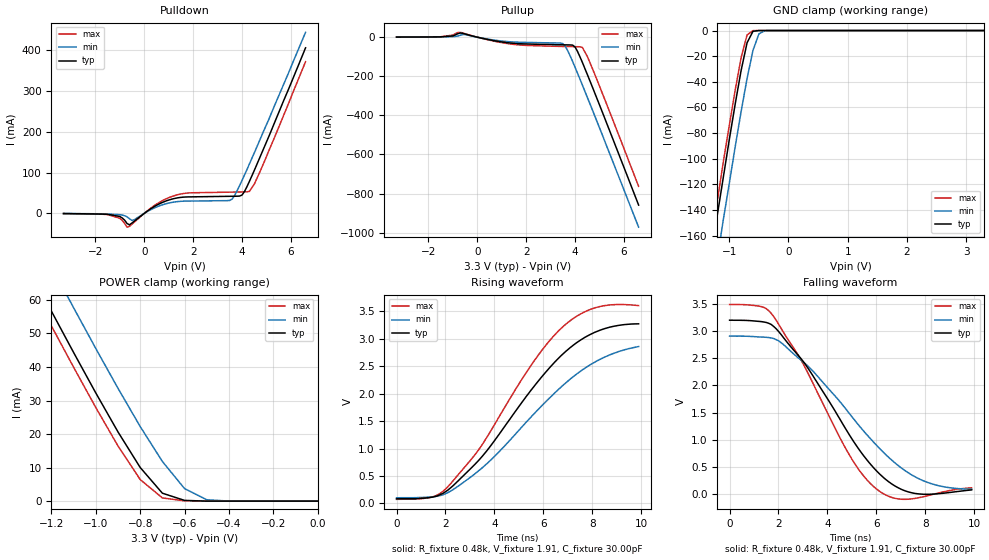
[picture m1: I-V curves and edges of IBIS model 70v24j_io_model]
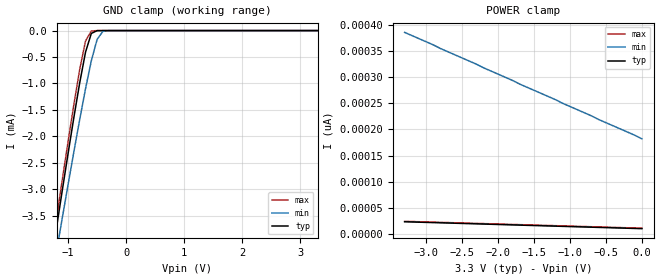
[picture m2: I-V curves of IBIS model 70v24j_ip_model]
| IBIS file 70v24j.ibs created by s2ibis2 version 1.0
| North Carolina State University Electronics Research Laboratory  1995
[IBIS ver]   2.1
[File name]   70v24j.ibs
[File Rev]   3.2
[Date]   11/11/04
[Source]   Integrated Device Technology, Inc.
[Notes]   1.Temperatures: typ=25C, min=100C, max=0C 2.Cemos7_5v process.
   3.RRmp rates based on 50 ohm load.
   IO & IP models corrected.  TH 11/11/04
[Disclaimer]   This information is for modeling purpose only, and is not
   guaranteed.
[Copyright]   Copyright 1997, Integrated Device Technology, Inc. all rights
   reserved
|   Component idt70v24
[Component]   idt70v24
[Manufacturer]   Integrated Device Technology
[Package]
| variable   typ   min   max
R_pkg   100.00m   50.00m   0.15
L_pkg   12.00nH   11.00nH   13.00nH
C_pkg   0.80pF   0.70pF   0.90pF
[Pin]  signal_name   model_name   R_pin   L_pin   C_pin
1   VCC   POWER
2   OEBL   70v24j_ip_model
3   IO0L   70v24j_io_model
4   IO1L   70v24j_io_model
5   GND   GND
6   IO2L   70v24j_io_model
7   IO3L   70v24j_io_model
8   IO4L   70v24j_io_model
9   IO5L   70v24j_io_model
10   IO6L   70v24j_io_model
11   IO7L   70v24j_io_model
12   IO8L   70v24j_io_model
13   IO9L   70v24j_io_model
14   IO10L   70v24j_io_model
15   IO11L   70v24j_io_model
16   IO12L   70v24j_io_model
17   IO13L   70v24j_io_model
18   GND   GND
19   IO14L   70v24j_io_model
20   IO15L   70v24j_io_model
21   VCC   POWER
22   GND   GND
23   IO0R   70v24j_io_model
24   IO1R   70v24j_io_model
25   IO2R   70v24j_io_model
26   VCC   POWER
27   IO3R   70v24j_io_model
28   IO4R   70v24j_io_model
29   IO5R   70v24j_io_model
30   IO6R   70v24j_io_model
31   IO7R   70v24j_io_model
32   IO8R   70v24j_io_model
33   IO9R   70v24j_io_model
34   IO10R   70v24j_io_model
35   IO11R   70v24j_io_model
36   IO12R   70v24j_io_model
37   IO13R   70v24j_io_model
38   IO14R   70v24j_io_model
39   GND   GND
40   IO15R   70v24j_io_model
41   OEBR   70v24j_ip_model
42   RWBR   70v24j_ip_model
43   GND   GND
44   SEMBR   70v24j_ip_model
45   CEBR   70v24j_ip_model
46   UBR   70v24j_ip_model
47   LBR   70v24j_ip_model
48   A12R   70v24j_ip_model
49   A11R   70v24j_ip_model
50   A10R   70v24j_ip_model
51   A9R   70v24j_ip_model
52   A8R   70v24j_ip_model
53   A7R   70v24j_ip_model
54   A6R   70v24j_ip_model
55   A5R   70v24j_ip_model
56   A4R   70v24j_ip_model
57   A3R   70v24j_ip_model
58   A2R   70v24j_ip_model
59   A1R   70v24j_ip_model
60   A0R   70v24j_ip_model
61   INTBR   70v24j_ip_model
62   BUSYBR   70v24j_io_model
63   MSBR   70v24j_ip_model
64   GND   GND
65   BUSYBL   70v24j_io_model
66   INTBL   70v24j_ip_model
67   A0L   70v24j_ip_model
68   A1L   70v24j_ip_model
69   A2L   70v24j_ip_model
70   A3L   70v24j_ip_model
71   A4L   70v24j_ip_model
72   A5L   70v24j_ip_model
73   A6L   70v24j_ip_model
74   A7L   70v24j_ip_model
75   A8L   70v24j_ip_model
76   A9L   70v24j_ip_model
77   A10L   70v24j_ip_model
78   A11L   70v24j_ip_model
79   A12L   70v24j_ip_model
80   LBL   70v24j_ip_model
81   UBL   70v24j_ip_model
82   CEBL   70v24j_ip_model
83   SEMBL   70v24j_ip_model
84   RWBL   70v24j_ip_model
| Models and submodels in the file (2): 70v24j_io_model (I/O), 70v24j_ip_model (Input)
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| in   in   dummy_model
| oel  oel   dummy_model
|   Model 70v24j_io_model
[Model]   70v24j_io_model
Model_type   I/O
Polarity   Non-Inverting
Enable   Active-High
Vinl =  0.800V
Vinh =  2.000V
Vmeas =  1.500V
C_comp   3.00pF   NA   NA
[Temperature Range]   25.00   100.00   0.000
[Voltage Range]   3.30V   3.00V   3.60V
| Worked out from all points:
|   slope of the pulldown table from 0 to 0.495 V, typ, clamps not added: 25.2 ohm
|   slope of the pullup table from 0 to 0.495 V, typ, clamps not added: 36.8 ohm
|   GND clamp passes 1 mA (typ) near -0.60 V on its own axis
|   POWER clamp passes 1 mA (typ) near -0.64 V on its own axis
|   rising waveform, R_fixture 0.48k, V_fixture 1.91, C_fixture 30.00pF: 20-80 % time 3.38ns typ, 3.7ns min, 3.12ns max; typ from 0.085 V to 3.27 V
|   falling waveform, R_fixture 0.48k, V_fixture 1.91, C_fixture 30.00pF: 20-80 % time 2.73ns typ, 3.33ns min, 2.38ns max; typ from 3.21 V to 0.072 V
[Pulldown]
| voltage   I(typ)   I(min)   I(max)
-3.3V     -300uA     -100uA     -400uA
-1.5V     -2.1mA     -1.4mA     -2.7mA
-1V       -7.34mA    -3mA       -11.82mA
-700mV    -24.76mA   -8.36mA    -33.61mA
-500mV    -23.52mA   -17.09mA   -26.24mA
400mV     16.4mA     13.1mA     18.68mA
1.2V      36.14mA    27.71mA    42.98mA
3.6V      42.09mA    35.54mA    52.29mA
4V        45.03mA    80.8mA     52.68mA
4.3V      78.13mA    121mA      54.03mA
4.5V      105mA      148mA      71.43mA
6.6V      406mA      444mA      372mA
[Pullup]
| voltage   I(typ)   I(min)   I(max)
-3.3V     500uA      600uA      600uA
-1.5V     1.64mA     1.1mA      1.95mA
-1V       6.29mA     2.68mA     10.62mA
-700mV    21.31mA    9.36mA     24.78mA
-500mV    16.4mA     13.61mA    17.88mA
1.3V      -29.2mA    -23.2mA    -33.88mA
3.5V      -39.14mA   -32.8mA    -47.46mA
3.7V      -39.55mA   -69.14mA   -47.96mA
4V        -50.05mA   -154mA     -48.63mA
4.3V      -129mA     -245mA     -52.79mA
4.5V      -190mA     -307mA     -97.94mA
6.6V      -859mA     -972mA     -763mA
[GND_clamp]
| voltage   I(typ)   I(min)   I(max)
-3.3V     -782mA     -813mA     -772mA
-1.3V     -172mA     -206mA     -161mA
-1.2V     -143mA     -177mA     -132mA
-1.1V     -114mA     -147mA     -102mA
-1V       -84.95mA   -119mA     -73.85mA
-900mV    -57.1mA    -90.38mA   -46.23mA
-800mV    -30.99mA   -63.03mA   -21.01mA
-700mV    -9.534mA   -37.37mA   -3.418mA
-600mV    -615uA     -15.47mA   -80.43uA
-500mV    -13.71uA   -2.616mA   -1.165uA
-400mV    -280nA     -145uA     -16.67nA
3.3V      38.75pA    737nA      37.71pA
[POWER_clamp]
| voltage   I(typ)   I(min)   I(max)
-3.3V     327mA      340mA      323mA
-1.3V     69.13mA    82.47mA    64.73mA
-1.2V     56.64mA    70mA       52.24mA
-1.1V     44.32mA    57.67mA    39.93mA
-1V       32.26mA    45.51mA    27.91mA
-900mV    20.65mA    33.65mA    16.46mA
-800mV    10.05mA    22.26mA    6.453mA
-700mV    2.37mA     11.84mA    958uA
-600mV    220uA      3.738mA    89.37uA
-500mV    1.528uA    408uA      130nA
-400mV    31.23nA    16.43uA    1.901nA
0V        38.73pA    1.793nA    42.34pA
[Ramp]
| variable   typ   min   max
dV/dt_r   0.97/2.56n   0.75/2.76n   1.16/2.41n
dV/dt_f   1.14/2.25n   0.88/2.68n   1.36/1.86n
R_load = 50.00
[Rising Waveform]
R_fixture = 0.48k
V_fixture = 1.91
C_fixture = 30.00pF
R_dut = 100.00m
L_dut = 4.00nH
C_dut = 10.00pF
| time   V(typ)   V(min)   V(max)
0s        84.6mV     104mV      75.61mV
1.4ns     111mV      119mV      112mV
2.1ns     244mV      197mV      306mV
3.4ns     806mV      611mV      1.005V
5.8ns     2.231V     1.716V     2.704V
6.4ns     2.541V     1.983V     3.037V
7ns       2.8V       2.226V     3.294V
7.6ns     2.997V     2.433V     3.469V
8.3ns     3.152V     2.62V      3.585V
9.9ns     3.272V     2.858V     3.604V
[Falling Waveform]
R_fixture = 0.48k
V_fixture = 1.91
C_fixture = 30.00pF
R_dut = 100.00m
L_dut = 4.00nH
C_dut = 10.00pF
| time   V(typ)   V(min)   V(max)
0s        3.205V     2.912V     3.495V
1.2ns     3.183V     2.896V     3.466V
1.7ns     3.127V     2.878V     3.333V
3.1ns     2.389V     2.401V     2.322V
5ns       1.016V     1.425V     641mV
6.1ns     382mV      854mV      57.18mV
6.8ns     135mV      557mV      -86.2mV
7.5ns     13.93mV    336mV      -90.56mV
8.5ns     126uV      155mV      10.6mV
9.9ns     71.96mV    85.36mV    111mV
|   Model 70v24j_ip_model
[Model]   70v24j_ip_model
Model_type   Input
Vinl =  0.800V
Vinh =  2.000V
Vmeas =  1.500V
C_comp   3.00pF   NA   NA
[Temperature Range]   25.00   100.00   0.000
[Voltage Range]   3.30V   3.00V   3.60V
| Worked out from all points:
|   GND clamp passes 1 mA (typ) near -0.80 V on its own axis
[GND_clamp]
| voltage   I(typ)   I(min)   I(max)
-3.3V     -19.14mA   -18.01mA   -19.55mA
-1.3V     -4.44mA    -4.817mA   -4.291mA
-1.2V     -3.724mA   -4.175mA   -3.549mA
-1.1V     -3.016mA   -3.537mA   -2.815mA
-900mV    -1.636mA   -2.286mA   -1.391mA
-800mV    -986uA     -1.68mA    -732uA
-700mV    -408uA     -1.1mA     -197uA
-600mV    -53.66uA   -571uA     -7.707uA
-500mV    -1.345uA   -166uA     -115nA
-400mV    -27.62nA   -13.71uA   -1.646nA
-200mV    -15.59pA   -29nA      -4.735pA
3.3V      9.916pA    201pA      9.6pA
[POWER_clamp]
| voltage   I(typ)   I(min)   I(max)
-3.3V     23.13pA    386pA      24pA
-2.3V     19.13pA    325pA      20pA
-2.2V     18.73pA    318pA      19.6pA
-1.2V     14.72pA    257pA      15.6pA
-1.1V     14.32pA    250pA      15.2pA
-100mV    10.32pA    189pA      11.2pA
0V        9.916pA    182pA      10.8pA
